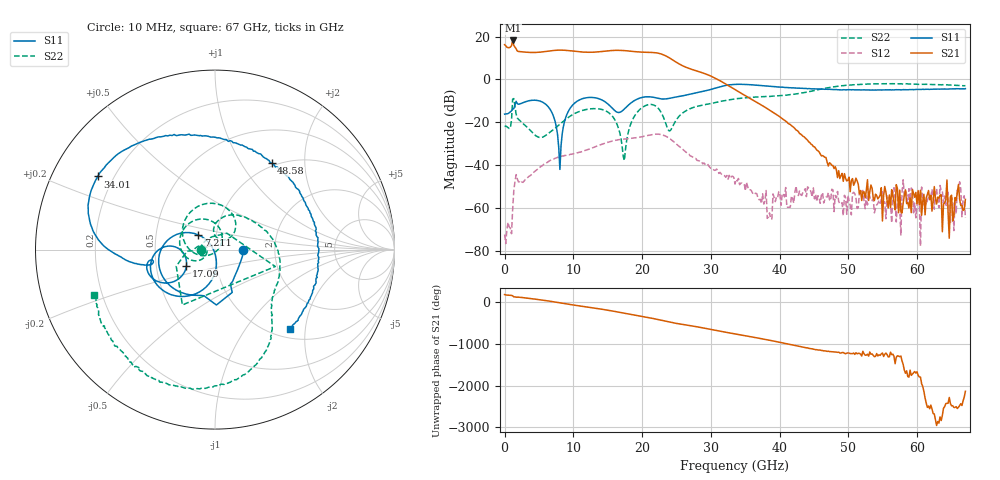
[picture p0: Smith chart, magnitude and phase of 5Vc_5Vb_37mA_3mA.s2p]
! MARKI MICROWAVE INC.
! Date:  05/05/2020
! Model Number:  APM-7099CH
! Description:  2-port Small Signal S-parameter data for APM-7099CH
! Frequency Range:  10 MHz to 67 GHz
! Port Configuration:  PORT 1: Input
!  PORT 2: Output
! Bias Condition: Vc = +5V, Vb = +5V
! APM-7099CH s2p files are only valid for small signal conditions (below -5 dBm input power)
!S2P File: Measurements: Mag<S11> Ang<S11>, Mag<S21> Ang<S21>, Mag<S12> Ang<S12>, Mag<S22> Ang<S22>!row 1
# Hz S  dB  R 50
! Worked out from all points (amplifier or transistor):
!   401 points, 10 MHz to 67 GHz, reference 50 ohm
!   highest |S21| = 18.2 dB at 1.182 GHz (marker M1)
!   |S21| within 3 dB of that: 872.9 MHz to 1.49 GHz (617.2 MHz wide, 52.2 % of centre)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
!   unconditionally stable (mu >= 1): start of sweep to end of sweep
!   at 11.06 GHz: K = 4.85, MAG = 13.5 dB, |S12| = -33.9 dB
!   at 33.51 GHz: K = 85.48, MAG = -0.3 dB, |S12| = -48.8 dB
!   at 67 GHz: K = 163475.80, MAG = -50.8 dB, |S12| = -64.6 dB
!   S11 on the Smith chart (normalised r, x): 10 MHz: 1.37, -0.00; 7.211 GHz: 0.82, +0.14; 17.09 GHz: 0.72, -0.13; 34.01 GHz: 0.14, +0.28; 48.58 GHz: 0.96, +1.37; 67 GHz: 1.18, -1.66
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1e7  -16.20 -0.1  16.21 178.7  -72.34 -58.6  -21.99 -179.0
1.182325e9  -13.84 -61.4  18.19 148.8  -60.49 88.2  -9.15 -15.7
1.68475e9  -10.21 -88.6  14.31 115.1  -44.40 -79.0  -16.15 -176.8
4.531825e9  -9.71 -160.0  12.60 66.9  -42.56 -167.0  -26.25 169.7
7.211425e9  -18.07 138.8  13.54 3.5  -37.02 129.3  -23.09 -145.3
9.3886e9  -14.21 -100.1  13.43 -55.8  -35.15 80.0  -17.46 -152.6
1.123082e10  -9.08 -134.6  12.81 -102.0  -33.69 46.0  -14.55 -178.4
1.458032e10  -10.35 179.0  13.21 175.8  -29.77 -22.0  -14.48 115.7
1.709245e10  -14.74 -150.2  13.53 102.3  -27.94 -85.6  -31.03 24.6
1.843225e10  -10.83 -142.0  13.15 62.4  -27.46 -119.0  -20.08 -163.2
2.0107e10  -8.30 -155.6  12.73 13.1  -26.67 -160.7  -12.89 140.7
2.127932e10  -8.16 -166.4  12.60 -23.8  -25.79 165.2  -11.67 99.4
2.245165e10  -8.91 -170.8  12.16 -65.2  -25.53 124.7  -13.85 56.9
2.379145e10  -8.91 -167.3  10.39 -114.4  -27.14 75.9  -23.46 53.9
2.496378e10  -8.18 -167.2  8.04 -151.3  -30.04 39.6  -18.88 94.1
2.848075e10  -5.87 -174.1  3.40 112.1  -38.36 -26.1  -12.17 47.0
3.3505e10  -2.31 152.7  -4.73 -43.4  -48.78 -97.4  -9.06 -1.3
3.400742e10  -2.28 148.0  -5.67 -58.0  -46.20 -95.8  -8.90 -5.8
4.472582e10  -4.36 79.0  -30.49 -40.5  -54.85 -42.3  -5.38 -53.7
4.857775e10  -4.81 56.8  -42.55 -119.5  -56.93 -61.6  -3.13 -73.5
5.594665e10  -4.79 12.2  -53.92 130.5  -55.52 -137.6  -2.01 -113.2
6.7e10  -4.31 -46.6  -55.98 23.1  -64.63 112.6  -2.88 -159.3
